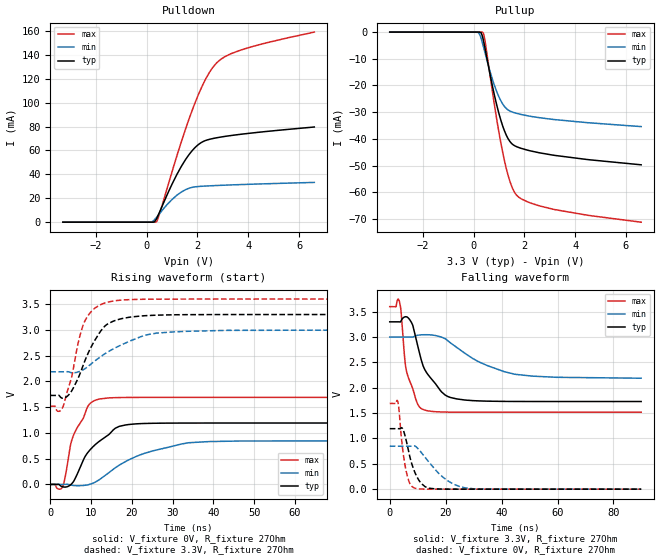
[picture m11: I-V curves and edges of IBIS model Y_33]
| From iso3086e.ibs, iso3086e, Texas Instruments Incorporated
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|   Y_33 Model
[Model]   Y_33
Model_type   3-state
|Signals   Y   positive pin
Polarity   Non-Inverting
Enable   Active-Low
Vmeas   = 1.56
Vref   = 1.65
Cref   = 50pF
|Rref = 27   |Note: 54 Ohm differential load;
| C_comp   obtained at 20MHz
|   typ   min   max
C_comp   99.04fF   99.46fF   109.8fF
[Voltage Range]   3.3   3   3.6
[Temperature Range]   40   125   -40
[Pullup Reference]   3.3   3   3.6
[Pulldown Reference]   0   0   0
[Power Clamp Reference]   3.3   3   3.6
[GND Clamp Reference]   0   0   0
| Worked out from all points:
|   slope of the pulldown table from 0 to 0.495 V, typ, clamps not added: 62.9 ohm
|   slope of the pullup table from 0 to 0.495 V, typ, clamps not added: 60.1 ohm
|   falling waveform, V_fixture 3.3V, R_fixture 27Ohm: 20-80 % time 7.52ns typ, 16.4ns min, 3.99ns max; typ from 3.3 V to 1.73 V
|   rising waveform, V_fixture 0V, R_fixture 27Ohm: 20-80 % time 7.28ns typ, 13.2ns min, 4.33ns max; typ from 0 V to 1.19 V
|   rising waveform, V_fixture 3.3V, R_fixture 27Ohm: 20-80 % time 5.73ns typ, 11ns min, 3.86ns max; typ from 1.73 V to 3.3 V
|   falling waveform, V_fixture 0V, R_fixture 27Ohm: 20-80 % time 3.86ns typ, 8.76ns min, 2.31ns max; typ from 1.19 V to 0 V
[Pulldown]
|   Voltage   I(typ)   I(min)   I(max)
-3.3V     -74.15pA   -201.6pA   -74.16pA
61.05mV   223nA      1.364uA    227.5nA
283.8mV   174uA      1.515mA    860.8nA
377.9mV   2.555mA    3.785mA    300.3uA
516.4mV   8.888mA    7.46mA     7.573mA
1.036V    33.45mA    19.73mA    44.85mA
1.605V    54.71mA    27.89mA    82.57mA
2.175V    66.94mA    30.06mA    113.3mA
2.67V     70.27mA    30.61mA    131.3mA
3.066V    71.73mA    30.97mA    138.3mA
3.709V    73.57mA    31.48mA    144.1mA
6.6V      79.65mA    33.28mA    159.1mA
[Pullup]
|   Voltage   I(typ)   I(min)   I(max)
-3.3V     145pA      164.8pA    166.6pA
179.9mV   -1.568uA   -131.2uA   -607nA
293.7mV   -271.7uA   -2.217mA   -1.786uA
363mV     -2.09mA    -4.547mA   -125.2uA
452.1mV   -6.116mA   -7.794mA   -3.35mA
793.6mV   -22.41mA   -19.16mA   -25.48mA
1.091V    -33.48mA   -25.99mA   -42.28mA
1.427V    -40.91mA   -29.54mA   -55.75mA
1.685V    -42.87mA   -30.41mA   -60.96mA
2.17V     -44.33mA   -31.43mA   -63.75mA
3.09V     -46.02mA   -32.66mA   -66.25mA
6.6V      -49.71mA   -35.4mA    -71.19mA
[Ramp]
R_load = 27
|   typ   min   max
dV/dt_r   0.71562/7.30721e-009  0.508619/1.30947e-008   1.01442/4.32636e-009
dV/dt_f   0.942998/7.53049e-009  0.487326/1.63914e-008   1.24939/4.00097e-009
[Falling Waveform]
V_fixture = 3.3V
V_fixture_min = 3V
V_fixture_max = 3.6V
R_fixture = 27Ohm
C_fixture = 0F
|   Time   V(typ)   V(min)   V(max)
0s        3.3V       3V         3.6V
3.36ns    3.3V       3V         3.721V
4ns       3.31V      3V         3.532V
5.96ns    3.399V     3V         2.338V
8.24ns    3.23V      2.999V     1.982V
11.88ns   2.44V      3.045V     1.573V
18.56ns   1.917V     2.998V     1.522V
23.92ns   1.78V      2.797V     1.518V
44.76ns   1.73V      2.266V     1.518V
89.92ns   1.728V     2.188V     1.518V
[Rising Waveform]
|Vcc
V_fixture = 0V
V_fixture_min = 0V
V_fixture_max = 0V
R_fixture = 27Ohm
C_fixture = 0F
|   Time   V(typ)   V(min)   V(max)
0s        -9.584uV   -22.99uV   -10.73uV
2.96ns    -45.58mV   -91.4uV    -54.51mV
3.72ns    -51.29mV   524uV      170.7mV
5.04ns    -3.692mV   -11.34mV   791.5mV
5.8ns     69.52mV    -21.68mV   973.9mV
9.4ns     638mV      -4.072mV   1.539V
11.84ns   826.4mV    82.62mV    1.654V
18.44ns   1.154V     443.3mV    1.689V
33.92ns   1.192V     808.9mV    1.691V
89.92ns   1.193V     847.7mV    1.691V
[Rising Waveform]
V_fixture = 3.3V
V_fixture_min = 3V
V_fixture_max = 3.6V
R_fixture = 27Ohm
C_fixture = 0F
|   Time   V(typ)   V(min)   V(max)
0s        1.728V     2.188V     1.518V
1.92ns    1.731V     2.188V     1.42V
2.96ns    1.674V     2.188V     1.481V
5.28ns    1.821V     2.169V     2.098V
6.88ns    2.073V     2.186V     2.759V
8.28ns    2.358V     2.237V     3.14V
10.52ns   2.743V     2.373V     3.396V
13.68ns   3.094V     2.552V     3.531V
26.16ns   3.288V     2.939V     3.598V
89.92ns   3.3V       3V         3.6V
[Falling Waveform]
|Gnd
V_fixture = 0V
V_fixture_min = 0V
V_fixture_max = 0V
R_fixture = 27Ohm
C_fixture = 0F
|   Time   V(typ)   V(min)   V(max)
0s        1.193V     847.7mV    1.691V
2.88ns    1.193V     847.7mV    1.725V
4.56ns    1.198V     847.7mV    821.1mV
5.72ns    999.3mV    847.7mV    400.6mV
7.16ns    648.6mV    847.5mV    116.2mV
8.92ns    340.7mV    851.4mV    21.26mV
13.68ns   23.71mV    557.2mV    191.8uV
21ns      406.5uV    156.5mV    101.8uV
27.2ns    -113.1uV   23.19mV    71.25uV
89.92ns   -9.584uV   -22.99uV   -10.73uV
